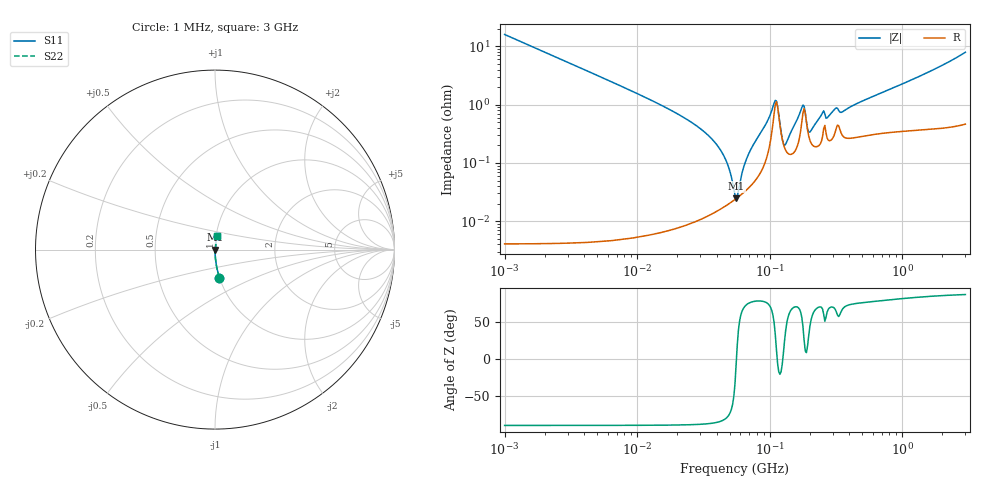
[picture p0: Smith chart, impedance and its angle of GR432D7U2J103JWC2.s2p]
!Murata Part Number: GR432D7U2J103JWC2
!These Parameters are Measured in Series Mode Connection
!Data Generated on Jun 10, 2025
!  o--ll--o
!Port1  Port2
!  o------o
!Operation Temp=25[degC], DC Bias Voltage=0[V]
!Freq. Start=1000[kHz] Stop=3[GHz] 401[Steps]
# Hz S RI R 50
!Freq.(Hz) S11(Real) S11(Imag) S21(Real) S21(Imag) S12(Real) S12(Imag) S22(Real) S22(Imag)
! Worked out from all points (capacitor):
!   401 points, 1 MHz to 3 GHz, reference 50 ohm
!   read as one part in series: C = 9.94 nF near 1.041 MHz
!   lowest |Z| = 24.7 mohm at 55.88 MHz (marker M1)
!   series resonance near 56.2 MHz, so ESL is about 810 pH
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1000000  0.025 -0.156  0.975 0.156  0.975 0.156  0.025 -0.156
3823119  0.00178 -0.0416  0.9982 0.0416  0.9982 0.0416  0.00178 -0.0416
1.461624e7  0.000168 -0.0102  0.9998 0.0102  0.9998 0.0102  0.000168 -0.0102
2.664524e7  0.000118 -0.00471  0.9999 0.00471  0.9999 0.00471  0.000118 -0.00471
3.820236e7  0.000146 -0.00232  0.9999 0.00232  0.9999 0.00232  0.000146 -0.00232
4.761141e7  0.00019 -0.000994  0.9998 0.000994  0.9998 0.000994  0.00019 -0.000994
5.477226e7  0.000236 -0.000156  0.9998 0.000156  0.9998 0.000156  0.000236 -0.000156
5.587962e7  0.000244 -3.43e-05  0.9998 3.43e-05  0.9998 3.43e-05  0.000244 -3.43e-05
6.826239e7  0.000361 0.00126  0.9996 -0.00126  0.9996 -0.00126  0.000361 0.00126
9.593103e7  0.00136 0.00497  0.9986 -0.00497  0.9986 -0.00497  0.00136 0.00497
1.081723e8  0.00716 0.00785  0.9928 -0.00785  0.9928 -0.00785  0.00716 0.00785
1.148668e8  0.00918 -0.00107  0.9908 0.00107  0.9908 0.00107  0.00918 -0.00107
1.244416e8  0.00256 -0.000345  0.9974 0.000345  0.9974 0.000345  0.00256 -0.000345
1.295243e8  0.00183 0.000819  0.9982 -0.000819  0.9982 -0.000819  0.00183 0.000819
1.748812e8  0.00504 0.00729  0.995 -0.00729  0.995 -0.00729  0.00504 0.00729
1.820241e8  0.00851 0.00393  0.9915 -0.00393  0.9915 -0.00393  0.00851 0.00393
1.971969e8  0.00289 0.00175  0.9971 -0.00175  0.9971 -0.00175  0.00289 0.00175
2.094008e8  0.00206 0.00327  0.9979 -0.00327  0.9979 -0.00327  0.00206 0.00327
2.507343e8  0.00287 0.00668  0.9971 -0.00668  0.9971 -0.00668  0.00287 0.00668
3.523638e8  0.00306 0.0068  0.9969 -0.0068  0.9969 -0.0068  0.00306 0.0068
8.005644e8  0.00363 0.0178  0.9964 -0.0178  0.9964 -0.0178  0.00363 0.0178
3e9  0.0108 0.0779  0.9892 -0.0779  0.9892 -0.0779  0.0108 0.0779
